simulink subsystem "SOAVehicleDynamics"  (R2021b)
settings: Solver=VariableStepAuto  StartTime=0.0  StopTime=10.0  RelTol=1e-3

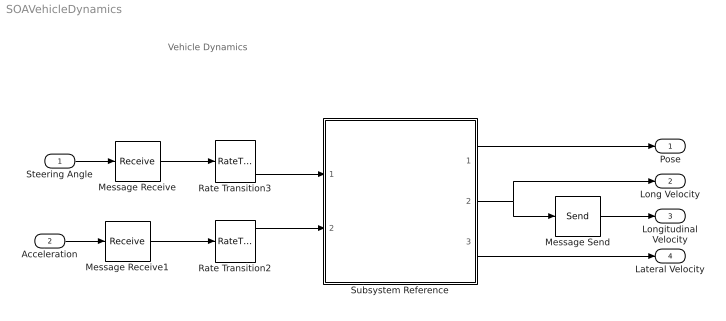
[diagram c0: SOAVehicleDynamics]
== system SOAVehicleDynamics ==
  note: Vehicle Dynamics
  Steering Angle : Inport  Unit=rad
  Acceleration : Inport  Port=2  Unit=m/s^2
  Message Receive : Receive  InputPortMessageModes=m
  Message Receive1 : Receive  InputPortMessageModes=m
  Message Send : Send  OutputPortMessageModes=m
  Rate Transition2 : RateTransition  OutPortSampleTime=Ts
  Rate Transition3 : RateTransition  OutPortSampleTime=Ts
  Subsystem Reference : Subsystem  ReferencedSubsystem=BicycleWithForceInput
  Pose : Outport  VectorParamsAs1DForOutWhenUnconnected=off
  Long Velocity : Outport  Port=2  Unit=m/s  SampleTime=0.1  VectorParamsAs1DForOutWhenUnconnected=off
  Longitudinal Velocity : Outport  Port=3
  Lateral Velocity : Outport  Port=4  Unit=m/s  SampleTime=0.1  VectorParamsAs1DForOutWhenUnconnected=off
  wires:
  Steering Angle/1 -> Message Receive/1
  Acceleration/1 -> Message Receive1/1
  Message Receive/1 -> Rate Transition3/1
  Message Receive1/1 -> Rate Transition2/1
  Message Send/1 -> Longitudinal Velocity/1
  Subsystem Reference/2 -> Message Send/1, Long Velocity/1
  Rate Transition3/1 -> Subsystem Reference/1
  Rate Transition2/1 -> Subsystem Reference/2
  Subsystem Reference/1 -> Pose/1
  Subsystem Reference/3 -> Lateral Velocity/1
